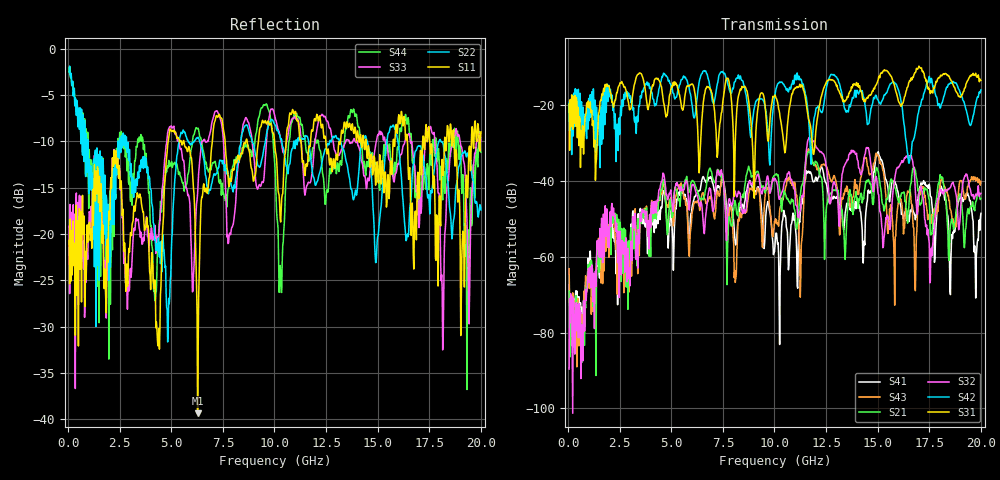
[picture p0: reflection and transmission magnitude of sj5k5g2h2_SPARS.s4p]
! FILE: E:\users\goganessyan\GBX_Backplane\FR408_backplane\1m_INBOUND_NEXT\sj5k5g2h2_SPARS.s4p
# MHZ S RI R 50.00
! FREQ  S11  S12  S13  S14
!  S21  S22  S23  S24
!  S31  S32  S33  S34
!  S41  S42  S43  S44
!  REAL  IMAG  REAL  IMAG  REAL  IMAG  REAL  IMAG
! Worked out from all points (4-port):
!   799 points, 50 MHz to 20 GHz, reference 50 ohm
!   strongest paths, dB at 50 MHz, 5.025 GHz, 10.03 GHz, 15.03 GHz, 20 GHz:
!     S31: -19.8, -14.9, -17.3, -13.3, -13.4
!     S42: -19.3, -15.3, -17.1, -18.6, -16.0
!     S32: -89.6, -45.1, -39.3, -43.4, -43.3
!     S21: -69.1, -49.6, -38.5, -37.4, -44.6
!     S43: -63.1, -47.2, -51.1, -33.2, -40.1
!     S41: -67.4, -50.8, -57.0, -32.3, -48.5
!   lowest |S11| = -39.3 dB at 6.275 GHz (marker M1), VSWR 1.02, Z = 51 + j0.503 ohm
!   |S11| at or under -10 dB: start of sweep to 4.851 GHz; 5.608 GHz to 6.989 GHz (1.381 GHz wide, 21.9 % of centre); 14.43 GHz to 15.75 GHz (1.312 GHz wide, 8.7 % of centre)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
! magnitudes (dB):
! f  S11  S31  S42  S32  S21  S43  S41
! 50 MHz  -20.7  -19.8  -19.3  -89.6  -69.1  -63.1  -67.4
! 4.85 GHz  -10.0  -20.2  -13.6  -44.2  -51.8  -47.0  -57.7
! 6.275 GHz  -39.3  -25.8  -16.8  -43.9  -42.7  -45.2  -42.9
! 7.25 GHz  -7.4  -32.7  -14.0  -37.1  -36.9  -42.5  -41.2
! 10.22 GHz  -15.8  -21.4  -14.0  -44.8  -41.3  -49.8  -71.3
! 11.62 GHz  -11.7  -22.9  -21.8  -29.1  -32.4  -31.8  -37.7
! 20 GHz  -9.0  -13.4  -16.0  -43.3  -44.6  -40.1  -48.5
